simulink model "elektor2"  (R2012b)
settings: Solver=ode45  StartTime=0.0  StopTime=1  RelTol=1e-3
undefined symbols (not defined in the file): A, constant, Ki, La, N, Ra, ray, Rc, T, Torque, U
libraries: powerlib x7, fl_lib x5, nesl_utility x3

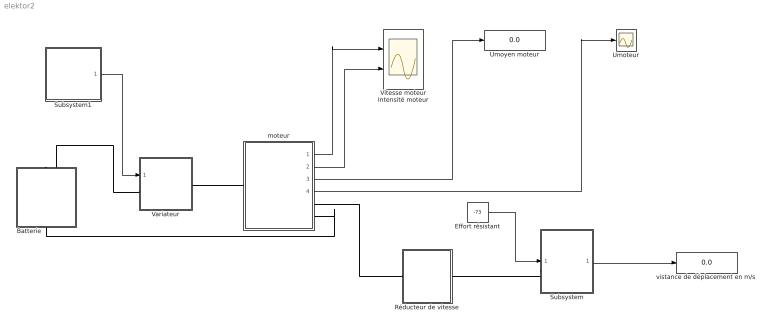
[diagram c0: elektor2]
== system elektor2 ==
  Batterie : Subsystem
  Effort résistant : Constant  Value=-73
  Réducteur de vitesse : Subsystem
  Subsystem : Subsystem
  Subsystem1 : Subsystem
  Umoteur : Scope
  Umoyen moteur : Display
  Variateur : Subsystem
  Vitesse moteur Intensité moteur : Scope  NumInputPorts=2
  moteur : Subsystem
  "vistance de déplacement en m/s " : Display
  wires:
  moteur/1(n moteur) -> Vitesse moteur Intensité moteur/1
  moteur/2(I moteur) -> Vitesse moteur Intensité moteur/2
  moteur/3(Umoyen moteur) -> Umoyen moteur/1
  moteur/4(Umoteur) -> Umoteur/1
  Effort résistant/1 -> Subsystem/1(force résistante)
  Subsystem/1(vitesse en m/s) -> "vistance de déplacement en m/s "/1
  Subsystem1/1(Signal) -> Variateur/1(générateur impulsions)
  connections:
  Variateur/RConn1 -- moteur/LConn1
  Réducteur de vitesse/LConn1 -- moteur/RConn1
  Subsystem/LConn1 -- Réducteur de vitesse/RConn1
  Variateur/LConn1 -- Batterie/RConn1
  Batterie/LConn1 -- moteur/RConn2

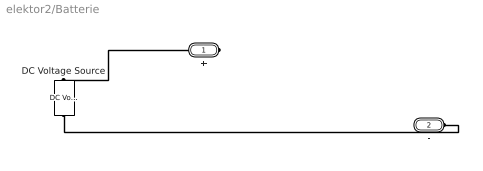
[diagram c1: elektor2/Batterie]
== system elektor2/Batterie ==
  DC Voltage Source : powerlib/Electrical Sources/DC Voltage Source  Amplitude=U  Measurements=None
  + : PMIOPort  Port=1  Side=Right
  - : PMIOPort  Port=2  Side=Left
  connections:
  +/RConn1 -- DC Voltage Source/RConn1
  DC Voltage Source/LConn1 -- -/RConn1

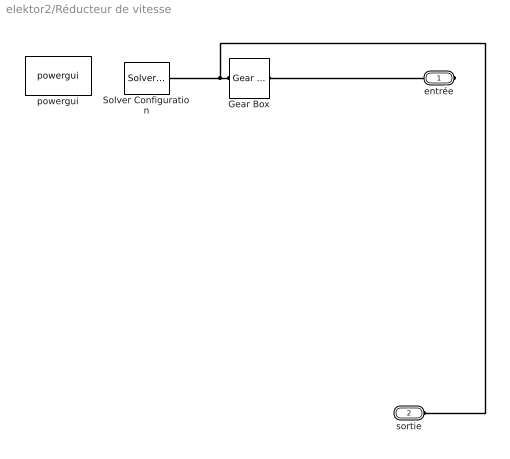
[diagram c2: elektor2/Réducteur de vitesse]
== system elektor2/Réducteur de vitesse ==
  Gear Box : fl_lib/Mechanical/Mechanisms/Gear Box  ratio=r  t_in_Log=off  t_out_Log=off  LocalVarNames=|t_in|t_out  LocalVarDescs=|t_in|t_out  LocalVarLogging=[0 0]
  Solver Configuration : nesl_utility/Solver Configuration  PhysicalDomain=network_engine_domain  LeftPortType=input  RightPortType=generic  SubClassName=solver  Accelerate=off  Profile=off  UseLocalSampling=off  FrequencyDomain=off  Tones=[]  Harmonics=[]  UseCCode=off  SimulateNoise=off  EnableSwitchedLinearOptims=on  DoDC=off  ResidualTolerance=1e-9  UseLocalSolver=off  LocalSolverChoice=NE_BACKWARD_EULER_ADVANCER  LocalSolverSampleTime=.001  DoFixedCost=off  MaxNonlinIter=3  MaxModeIter=2  LinearAlgebra=Sparse  DelaysMemoryBudget=1024
  powergui : powerlib/powergui  Priority=1  SimulationMode=Continuous  SolverType=Tustin  SampleTime=50e-6  frequency=60  SPID=off  DisableSnubberDevices=off  DisableRonSwitches=off  DisableVfSwitches=off  SwTol=0  Interpol=off  DisplayEquations=off  FunctionMessages=off  frequencyindice=0  Pbase=100e6  ErrMax=1e-4  Iterations=50  UnitsV=kV  UnitsW=MW  echomessages=off  HookPort=off  EnableUseOfTLC=off  x0status=blocks  RestoreLinks=warning  ResistiveCurrentMeasurement=off  Ylog=off  Xlog=on  ShowGrid=off  save=off  variable=ZData  ZoomFFT=off  StartTime=0.0  cycles=1  DisplayStyle=1  FreqAxis=off  MaxFrequency=1000  frequencyindicesteady=1  display=off  methode=off
  entrée : PMIOPort  Port=1  Side=Right
  sortie : PMIOPort  Port=2  Side=Left
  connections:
  entrée/RConn1 -- Gear Box/RConn1
  Gear Box/LConn1 -- sortie/RConn1 -- Solver Configuration/RConn1

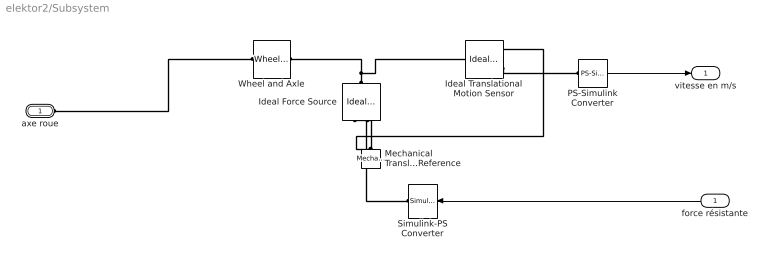
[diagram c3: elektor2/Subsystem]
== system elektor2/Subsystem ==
  force résistante : Inport
  Ideal Force Source : fl_lib/Mechanical/Mechanical Sources/Ideal Force Source  v_Log=off  f_Log=off  LocalVarNames=|v|f  LocalVarDescs=|v|f  LocalVarLogging=[0 0]
  Ideal Translational Motion Sensor : fl_lib/Mechanical/Mechanical Sensors/Ideal Translational Motion Sensor  offset=0 m  v_Log=off  f_Log=off  x_Log=off  LocalVarNames=|v|f|x  LocalVarDescs=|v|f|x  LocalVarLogging=[0 0 0]
  Mechanical Translational Reference : fl_lib/Mechanical/Translational Elements/Mechanical Translational Reference  f_Log=off  LocalVarNames=|f  LocalVarDescs=|f  LocalVarLogging=0
  PS-Simulink Converter : nesl_utility/PS-Simulink Converter  PhysicalDomain=network_engine_domain  LeftPortType=input  RightPortType=output  SubClassName=ps_output  PseudoPeriodic=off  Frequencies=[]  Unit=1  AffineConversion=off
  Simulink-PS Converter : nesl_utility/Simulink-PS Converter  PhysicalDomain=network_engine_domain  LeftPortType=input  RightPortType=output  SubClassName=ps_input  PseudoPeriodic=off  Frequencies=[]  NoiseDistribution=none  NoiseParameters=[]  Unit=1  AffineConversion=off  InputFilterTimeConstant=.001  UdotUserProvided=[]  SimscapeFilterOrder=1  InputFiltering=off
  Wheel and Axle : fl_lib/Mechanical/Mechanisms/Wheel and Axle  R=ray m  or=1  orient=1  t_Log=off  f_Log=off  LocalVarNames=|t|f  LocalVarDescs=|t|f  LocalVarLogging=[0 0]
  axe roue : PMIOPort  Port=1  Side=Left
  vitesse en m/s : Outport
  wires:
  force résistante/1 -> Simulink-PS Converter/1
  PS-Simulink Converter/1 -> vitesse en m/s/1
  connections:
  Ideal Force Source/LConn1 -- Ideal Translational Motion Sensor/LConn1 -- Wheel and Axle/RConn1
  Mechanical Translational Reference/LConn1 -- Ideal Translational Motion Sensor/RConn1 -- Ideal Force Source/RConn2
  Simulink-PS Converter/RConn1 -- Ideal Force Source/RConn1
  Ideal Translational Motion Sensor/RConn3 -- PS-Simulink Converter/LConn1
  Wheel and Axle/LConn1 -- axe roue/RConn1

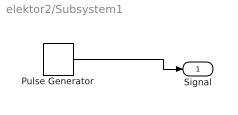
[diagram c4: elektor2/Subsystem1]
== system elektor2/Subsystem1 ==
  Pulse Generator : DiscretePulseGenerator  PulseType=Time based  Amplitude=5  Period=T  PulseWidth=Rc
  Signal : Outport
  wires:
  Pulse Generator/1 -> Signal/1

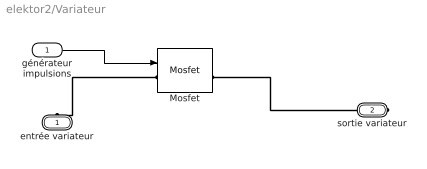
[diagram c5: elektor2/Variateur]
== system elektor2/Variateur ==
  générateur impulsions : Inport
  Mosfet : powerlib/Power Electronics/Mosfet  Ron=0.1  Lon=0  Rd=0.01  Vfd=0  IC=0  Rs=1e5  Cs=inf  Measurements=on
  entrée variateur : PMIOPort  Port=1  Side=Left
  sortie variateur : PMIOPort  Port=2  Side=Right
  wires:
  générateur impulsions/1 -> Mosfet/1
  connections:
  Mosfet/LConn1 -- entrée variateur/RConn1
  Mosfet/RConn1 -- sortie variateur/RConn1

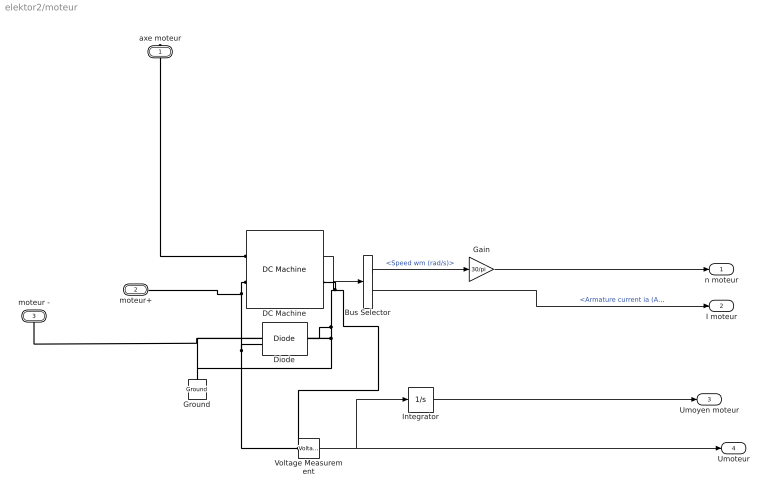
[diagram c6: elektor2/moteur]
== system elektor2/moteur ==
  Bus Selector : BusSelector  OutputSignals=Speed wm (rad/s),Armature current ia (A)
  DC Machine : powerlib/Machines/DC Machine  PresetModel=No  MechanicalLoad=Mechanical rotational port  FieldType=Permanent magnet  ShowDetailedParameters=on  RLa="[ Ra  La]"  RLf="[ 240  120]"  Laf=1.8  MachineConstant=Torque constant (N.m/A)  Ke=0.0744  Kt=Ki  J=0.001  Bm=0.00001  Tf=0.00001  w0=0  Ifinit=1  TsPowergui=0  TsBlock=-1
  Diode : powerlib/Power Electronics/Diode  Ron=0.001  Lon=0  Vf=0.8  IC=0  UseSnubber=off  Rs=500  Cs=250e-9  Measurements=on
  Gain : Gain  Gain=30/pi
  Ground : powerlib/Elements/Ground  LConnTagsString=a
  Integrator : Integrator
  Voltage Measurement : powerlib/Measurements/Voltage Measurement  PhasorSimulation=off  OutputType=Complex  PSBequivalent=0
  axe moteur : PMIOPort  Port=1  Side=Right
  moteur+ : PMIOPort  Port=2  Side=Left
  moteur - : PMIOPort  Port=3  Side=Right
  n moteur : Outport
  I moteur : Outport  Port=2
  Umoyen moteur : Outport  Port=3
  Umoteur : Outport  Port=4
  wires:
  DC Machine/1 -> Bus Selector/1
  Bus Selector/2 -> I moteur/1  "<Armature current ia (A)>"
  Bus Selector/1 -> Gain/1  "<Speed wm (rad/s)>"
  Gain/1 -> n moteur/1
  Voltage Measurement/1 -> Umoteur/1, Integrator/1
  Integrator/1 -> Umoyen moteur/1
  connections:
  DC Machine/RConn1 -- Diode/LConn1 -- moteur -/RConn1 -- Ground/LConn1 -- Voltage Measurement/LConn2
  Voltage Measurement/LConn1 -- moteur+/RConn1 -- DC Machine/LConn2 -- Diode/RConn1
  axe moteur/RConn1 -- DC Machine/LConn1
